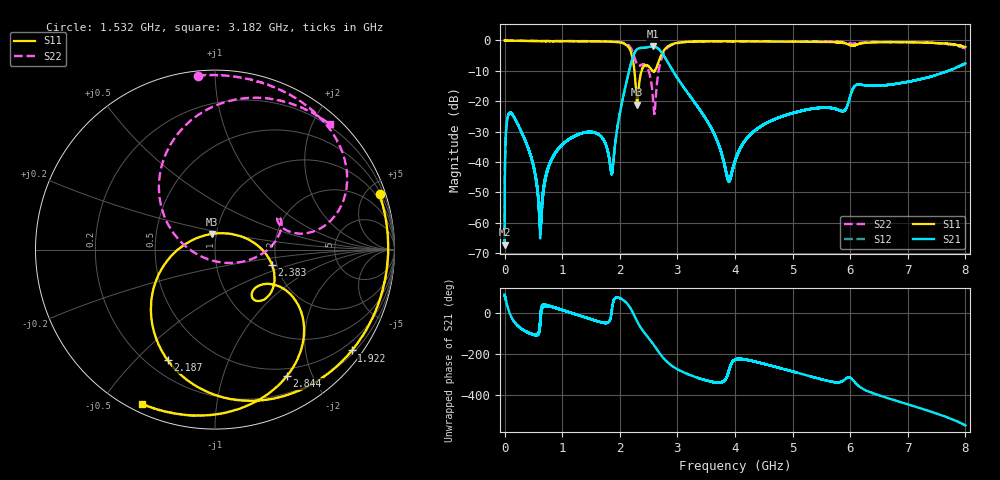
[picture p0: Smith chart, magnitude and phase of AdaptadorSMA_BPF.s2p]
#  HZ  S  DB  R  50.00
! Rohde & Schwarz ZVA/B
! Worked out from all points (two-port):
!   30000 points, 300 kHz to 8 GHz, reference 50 ohm
!   highest |S21| = -1.96 dB at 2.579 GHz (marker M1); lowest = -67.2 dB at 300 kHz (marker M2)
!   |S21| within 3 dB of the highest: 2.236 GHz to 2.763 GHz (526.9 MHz wide, 21.1 % of centre)
!   lowest |S11| = -21.1 dB at 2.301 GHz (marker M3), VSWR 1.19, Z = 47.7 + j8.35 ohm
!   |S11| at or under -10 dB: 2.254 GHz to 2.377 GHz (123.3 MHz wide, 5.33 % of centre); 2.569 GHz to 2.607 GHz (37.75 MHz wide, 1.46 % of centre)
!   |S22| runs from -24.2 to 0.0 dB; largest |S21 - S12| = 0.0026
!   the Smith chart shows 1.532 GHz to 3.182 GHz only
!   S11 on the Smith chart (normalised r, x): 1.532 GHz: 0.62, +6.02; 1.922 GHz: 0.28, -3.02; 2.187 GHz: 0.28, -0.62; 2.383 GHz: 1.89, -0.35; 2.844 GHz: 0.40, -1.65; 3.182 GHz: 0.04, -0.63
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300000  0.00 -0.4  -67.21 90.1  -67.72 91.1  -0.00 -0.4
6.829972e7  -0.04 -77.1  -24.19 15.1  -24.20 15.0  -0.04 -72.3
3.040321e8  -0.13 -177.5  -30.57 -78.6  -30.60 -78.8  -0.11 -161.1
6.221641e8  -0.21 130.2  -63.35 -62.6  -59.68 -23.9  -0.14 162.2
8.274966e8  -0.24 103.6  -38.66 29.2  -38.84 29.9  -0.17 145.7
1.333628e9  -0.27 42.9  -30.50 -15.1  -30.56 -15.1  -0.19 109.5
1.532027e9  -0.28 18.7  -30.19 -33.0  -30.15 -32.8  -0.22 95.6
1.921892e9  -0.47 -36.4  -33.72 73.0  -33.68 73.7  -0.39 62.7
2.187224e9  -3.48 -113.2  -8.03 23.4  -8.02 23.3  -2.32 20.9
2.300824e9  -21.09 100.2  -2.87 -39.7  -2.87 -39.8  -7.92 16.8
2.382957e9  -9.68 -14.8  -2.43 -78.5  -2.44 -78.5  -7.95 26.9
2.579489e9  -10.14 -46.9  -1.96 -150.5  -1.97 -150.5  -19.66 -45.6
2.666956e9  -7.38 -29.7  -2.66 174.4  -2.66 174.4  -10.79 152.7
2.844288e9  -1.83 -60.3  -7.52 117.0  -7.52 116.9  -2.15 93.1
3.181887e9  -0.44 -115.3  -17.35 63.0  -17.33 62.9  -0.47 47.4
4.000283e9  -0.27 148.2  -39.82 133.4  -39.78 133.6  -0.25 -8.7
4.633881e9  -0.33 80.6  -26.42 103.9  -26.39 104.1  -0.23 -44.3
5.333611e9  -0.40 7.6  -22.47 50.6  -22.49 50.8  -0.28 -83.2
5.907475e9  -0.91 -56.2  -22.96 36.7  -22.99 36.9  -0.60 -116.8
6.666939e9  -0.55 -131.0  -14.59 -54.8  -14.59 -54.8  -0.51 -155.6
7.277336e9  -0.69 164.3  -12.48 -108.0  -12.48 -108.1  -0.70 167.4
8e9  -2.13 85.9  -7.56 173.7  -7.54 173.7  -2.62 115.1
